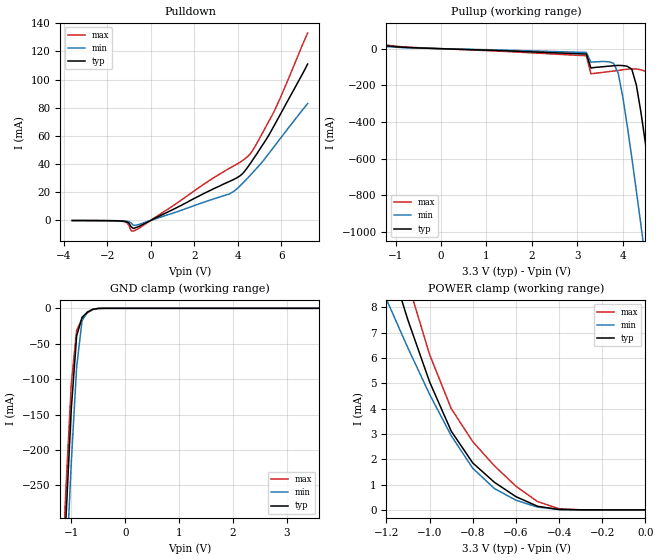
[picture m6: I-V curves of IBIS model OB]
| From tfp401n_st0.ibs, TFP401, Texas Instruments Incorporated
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|   OUTPUT  MODEL
[Model]   OB
Model_type   3-state
| variable   typ   min   max
C_comp   2pF   NA   NA
|   typ   min   max
[Temperature Range]   25.0   70   0
[Voltage range]   3.3V   3.0V   3.6V
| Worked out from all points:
|   slope of the pulldown table from 0 to 0.495 V, typ, clamps not added: 130 ohm
|   slope of the pullup table from 0 to 0.495 V, typ, clamps not added: 124 ohm
|   GND clamp passes 1 mA (typ) near -0.57 V on its own axis
|   POWER clamp passes 1 mA (typ) near -0.68 V on its own axis
[GND_clamp]
|Voltage   I(typ)   I(min)   I(max)
-3.6V     -5.15A     -5.23A     -5.11A
-1.2V     -475mA     -560mA     -430mA
-1.1V     -300mA     -383mA     -257mA
-1V       -143mA     -219mA     -108mA
-900mV    -39mA      -83.1mA    -31.1mA
-800mV    -12.8mA    -17.6mA    -15mA
-700mV    -5.33mA    -5.31mA    -6.46mA
-600mV    -1.35mA    -1.53mA    -1.56mA
-400mV    -9.01uA    -20.2uA    -7.51uA
3.6V      729nA      380uA      131pA
[Power_clamp]
|Note that the [Power_clamp] voltage table is referenced to Vcc
|and is calculated using Vtable=Vcc-Vmeasured.
|Voltage   I(typ)   I(min)   I(max)
-3.3V     74.5mA     52.3mA     96.8mA
-1.2V     10.2mA     8.31mA     12.3mA
-1.1V     7.48mA     6.38mA     8.95mA
-1V       5.05mA     4.56mA     6.13mA
-900mV    3.11mA     2.93mA     4mA
-800mV    1.85mA     1.64mA     2.69mA
-700mV    1.09mA     842uA      1.74mA
-600mV    520uA      380uA      933uA
-500mV    142uA      107uA      326uA
-400mV    14.4uA     13.6uA     43.6uA
-300mV    729nA      1.02uA     2.09uA
0V        124pA      197pA      131pA
[Pulldown]
|Voltage   I(typ)   I(min)   I(max)
-3.6V     -61.5uA    -42.8uA    -79.2uA
-1.3V     -473uA     -291uA     -661uA
-1.1V     -993uA     -538uA     -1.54mA
-1V       -1.9mA     -876uA     -3.36mA
-900mV    -4.47mA    -1.78mA    -7.33mA
-800mV    -5.66mA    -3.31mA    -7.6mA
3.6V      27.6mA     18.6mA     36.9mA
4.1V      31.7mA     24.6mA     41.3mA
4.4V      36.7mA     29.3mA     44.7mA
4.8V      45.7mA     36mA       52.8mA
5.7V      68.3mA     53.1mA     78.6mA
7.2V      111mA      83mA       133mA
[Pullup]
|Note that the [Pullup] voltage table is referenced to Vcc
|and is calculated using Vtable=Vcc-Vmeasured.
|Voltage   I(typ)   I(min)   I(max)
-3.3V     76.3mA     53.8mA     99mA
3.2V      -29.3mA    -20.5mA    -38.6mA
3.3V      -105mA     -73.4mA    -137mA
3.8V      -92.9mA    -79.6mA    -122mA
4V        -92.1mA    -261mA     -115mA
4.2V      -112mA     -595mA     -110mA
4.4V      -346mA     -960mA     -115mA
4.5V      -516mA     -1.15A     -123mA
4.6V      -694mA     -1.33A     -174mA
4.8V      -1.06A     -1.71A     -471mA
5.1V      -1.63A     -2.29A     -1.01A
6.6V      -4.56A     -5.23A     -3.92A
[Ramp]
|   typ   min   max
dV/dt_r   2.03v/1.1ns   1.97/2ns   1.94v/600ps
dV/dt_f   2.02v/900ps   1.8v/1.4ns   1.88v/500ps
R_load = 5K
